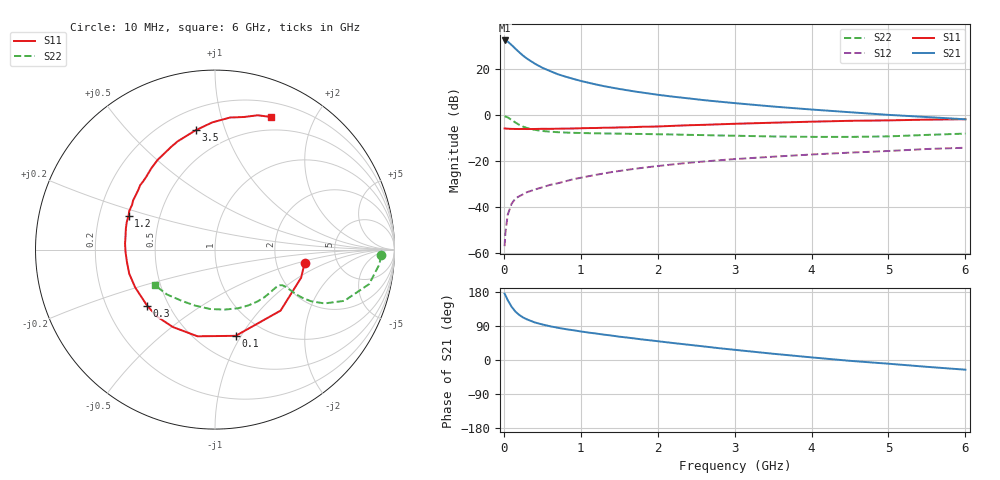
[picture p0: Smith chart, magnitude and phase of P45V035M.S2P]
! SIEMENS Small Signal Semiconductors
! BFP182
! Si NPN RF Bipolar Junction Transistor in SOT143
! VCE = 5 V  IC = 35 mA
! Common Emitter S-Parameters:  March  1996
# GHz  S  MA  R  50
!  f  S11  S21  S12  S22
! GHz  MAG  ANG  MAG  ANG  MAG  ANG  MAG  ANG
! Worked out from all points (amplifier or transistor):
!   36 points, 10 MHz to 6 GHz, reference 50 ohm
!   highest |S21| = 32.3 dB at 10 MHz (marker M1)
!   |S21| within 3 dB of that: start of sweep to 132.5 MHz
!   unconditionally stable (mu >= 1): start of sweep to 10.07 MHz; 491.4 MHz to 5.688 GHz
!   at 250 MHz: K = 0.68, MSG = 30.1 dB, |S12| = -34.5 dB
!   at 1.4 GHz: K = 1.28, MAG = 15.2 dB, |S12| = -24.9 dB
!   at 6 GHz: K = 0.98, MSG = 6.2 dB, |S12| = -14.3 dB
!   S11 on the Smith chart (normalised r, x): 10 MHz: 2.90, -0.59; 100 MHz: 0.75, -0.95; 300 MHz: 0.38, -0.31; 1.2 GHz: 0.33, +0.17; 3.5 GHz: 0.33, +0.80; 6 GHz: 0.35, +1.45
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0.01  0.5048 -8.7  41.23 175.1  0.0014 79.5  0.9244 -2.0
0.02  0.5047 -18.1  41.05 171.2  0.0027 77.4  0.9203 -5.0
0.05  0.4991 -42.9  39.08 158.2  0.0067 77.0  0.8802 -12.6
0.1  0.4941 -76.5  32.95 140.7  0.0116 59.9  0.7753 -21.6
0.15  0.4927 -101.4  27.35 127.9  0.0152 55.8  0.6795 -26.2
0.2  0.4911 -118.6  22.85 118.9  0.017 53.4  0.6065 -28.3
0.25  0.4936 -130.9  19.32 112.3  0.0188 51.8  0.5544 -28.9
0.3  0.4904 -140.5  16.66 107.3  0.0208 51.6  0.5174 -28.8
0.4  0.4922 -154.7  13 99.3  0.0237 53.1  0.4718 -28.2
0.5  0.4964 -164.4  10.54 93.8  0.0266 53.7  0.4458 -27.8
0.6  0.4955 -172.3  8.926 89.1  0.03 55.4  0.4298 -27.8
0.7  0.4985 -178.3  7.633 85.1  0.0325 57.0  0.4193 -28.2
0.8  0.5023 176.1  6.761 81.6  0.0359 57.5  0.412 -28.8
1.1  0.5151 162.7  4.976 72.4  0.0463 58.4  0.3991 -32.0
1.2  0.5169 158.8  4.554 69.8  0.0497 57.9  0.3963 -33.3
1.7  0.542 141.9  3.213 56.8  0.0671 56.2  0.3847 -41.2
2.2  0.5753 128.1  2.477 44.8  0.0838 52.6  0.3738 -50.6
2.8  0.622 113.2  1.932 31.1  0.1029 47.1  0.3557 -63.7
3.5  0.6736 99.2  1.513 16.5  0.123 40.9  0.3384 -81.3
4.5  0.7406 83.5  1.137 -2.2  0.1509 32.1  0.331 -109.4
5.5  0.7851 72.4  0.894 -18.0  0.1808 23.7  0.3661 -136.9
6  0.8018 67.2  0.799 -25.6  0.1926 18.5  0.3904 -149.7
